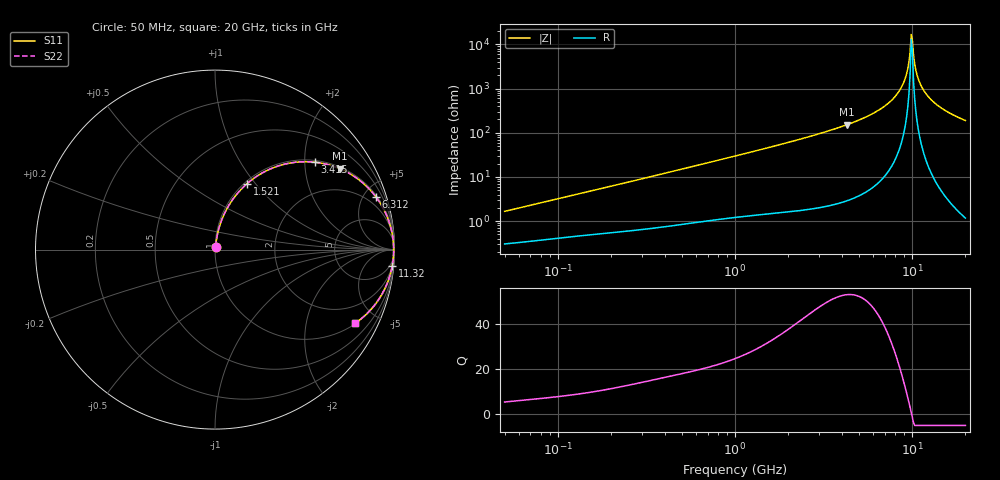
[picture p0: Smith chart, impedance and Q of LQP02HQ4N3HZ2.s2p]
!Murata Part Number: LQP02HQ4N3HZ2
!These Parameters are Measured in Series Mode Connection
!  o--[Z]--o
!Port1  Port2
!  o-------o
!Freq. Start=50[MHz] Stop=20[GHz], 401[Steps]
# Hz S RI R 50
!Freq.(Hz) S11(Real) S11(Imag) S21(Real) S21(Imag) S12(Real) S12(Imag) S22(Real) S22(Imag)
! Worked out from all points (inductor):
!   401 points, 50 MHz to 20 GHz, reference 50 ohm
!   read as one part in series: L = 5.15 nH near 51.52 MHz
!   highest Q = 52.8 at 4.276 GHz (marker M1), where L = 5.65 nH
!   self-resonance near 9.892 GHz
!   S11 on the Smith chart (normalised r, x): 50 MHz: 1.01, +0.03; 1.521 GHz: 1.03, +0.91; 3.415 GHz: 1.04, +2.24; 6.312 GHz: 1.14, +6.11; 11.32 GHz: 2, -22; 20 GHz: 1.02, -3.80
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5e7  0.0033 0.0162  0.9967 -0.0162  0.9967 -0.0162  0.0033 0.0162
1.364002e8  0.00644 0.0421  0.9936 -0.0421  0.9936 -0.0421  0.00644 0.0421
3.721004e8  0.0193 0.1093  0.9807 -0.1093  0.9807 -0.1093  0.0193 0.1093
1e9  0.0902 0.2668  0.9098 -0.2668  0.9098 -0.2668  0.0902 0.2668
1.521052e9  0.1787 0.3676  0.8213 -0.3676  0.8213 -0.3676  0.1787 0.3676
2.728004e9  0.424 0.4833  0.576 -0.4833  0.576 -0.4833  0.424 0.4833
3.415248e9  0.5558 0.487  0.4442 -0.487  0.4442 -0.487  0.5558 0.487
4.275624e9  0.6938 0.4515  0.3062 -0.4515  0.3062 -0.4515  0.6938 0.4515
6.311513e9  0.898 0.2918  0.102 -0.2918  0.102 -0.2918  0.898 0.2918
7.442007e9  0.9545 0.1941  0.0455 -0.1941  0.0455 -0.1941  0.9545 0.1941
8.264682e9  0.9784 0.126  0.0216 -0.126  0.0216 -0.126  0.9784 0.126
8.907419e9  0.9892 0.0756  0.0108 -0.0756  0.0108 -0.0756  0.9892 0.0756
9.316812e9  0.9931 0.0449  0.00688 -0.0449  0.00688 -0.0449  0.9931 0.0449
9.745021e9  0.9951 0.014  0.00487 -0.014  0.00487 -0.014  0.9951 0.014
9.892087e9  0.9954 0.00368  0.00463 -0.00368  0.00463 -0.00368  0.9954 0.00368
1.019291e10  0.9952 -0.017  0.0048 0.017  0.0048 0.017  0.9952 -0.017
1.050288e10  0.9942 -0.0376  0.00583 0.0376  0.00583 0.0376  0.9942 -0.0376
1.066139e10  0.9933 -0.0479  0.00667 0.0479  0.00667 0.0479  0.9933 -0.0479
1.131968e10  0.9878 -0.0889  0.0122 0.0889  0.0122 0.0889  0.9878 -0.0889
1.238412e10  0.9732 -0.1492  0.0268 0.1492  0.0268 0.1492  0.9732 -0.1492
1.396067e10  0.9422 -0.2259  0.0578 0.2259  0.0578 0.2259  0.9422 -0.2259
2e10  0.7813 -0.4103  0.2187 0.4103  0.2187 0.4103  0.7813 -0.4103
